FUNCTION_BLOCK ConfigurationManager

(* --------------------------------------------- *)
(* Triamec Motion AG, 6340 Baar, Switzerland     *)
(* Sample Code may be adapted to customer need   *)
(* --------------------------------------------- *)

(* Trialink Configuration *)
gTrialink.Config.nDevId := 1; (* DPRAM id, see TwinCatSystemManager *)
//Trialink.Config.RootFolder := 'C:\Machine\'; (* for debugging *)
gTrialink.Config.TcEventEnable := TRUE;
//gTrialink.Config.FastFilterFrequency := 200; (* deprecated *)

(* scale between Nci and PLC *)
	gCncAxes[1].inc_per_unit   := 1000000;
	gCncAxes[2].inc_per_unit   := 1000000;

(* define the axis parameters *)
(* ---------- Axis 1 ------------------------------------------------------------------ *)
	gAxes[1].Config.Simulate   := FALSE;
	gAxes[1].Config.Station    := 10; (* The drive address *)
	gAxes[1].Config.SubAxis    := TL_Config.SubAxis.FirstAxis; (* first or second axis of a two axes drive *)
	gAxes[1].Config.GearFactor := 1;  (* multiplication factor of position and velocity data *)
	gAxes[1].Config.ModuloWrap := 0;  (* modulo wrap for rotation axes *)
	
(* ---------- Axis 2 ------------------------------------------------------------------ *)
	gAxes[2].Config.Simulate   := TRUE;
	gAxes[2].Config.Station    := 10; (* The drive address *)
	gAxes[2].Config.SubAxis    := TL_Config.SubAxis.SecondAxis; (* first or second axis of a two axes drive *)
	gAxes[2].Config.GearFactor := 1;  (* multiplication factor of position and velocity data *)
	gAxes[2].Config.ModuloWrap := 0;  (* modulo wrap for rotation axes *)

END_FUNCTION_BLOCK
